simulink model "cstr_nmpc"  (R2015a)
settings: Solver=ode15s  StartTime=0.0  StopTime=5  RelTol=1e-5
StopFcn:
  | plot_reactor
undefined symbols (not defined in the file or in its folder): nmpc
libraries: simulink x4

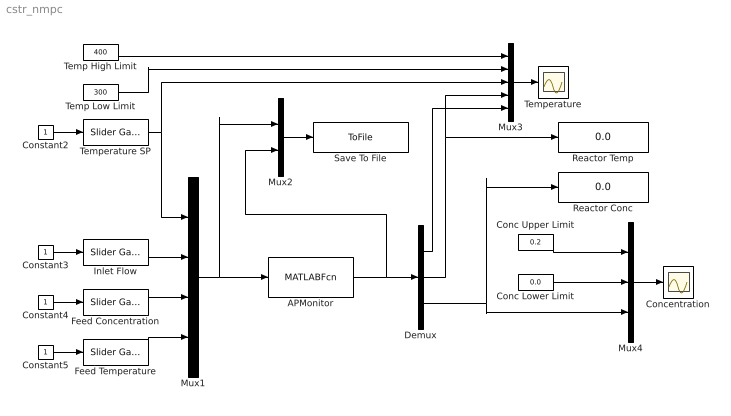
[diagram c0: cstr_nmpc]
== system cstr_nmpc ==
  APMonitor : MATLABFcn  MATLABFcn=nmpc(u)  OutputDimensions=3  SampleTime=0.05
  Conc Lower Limit : Constant  Value=0.0
  Conc Upper Limit : Constant  Value=0.2
  Concentration : Scope
  Constant{2..5} (4 alike) : Constant
  Demux : Demux  Outputs=3
  Feed Concentration : simulink/Math Operations/Slider Gain  low=0  gain=1  high=1
  Feed Temperature : simulink/Math Operations/Slider Gain  low=300  gain=350  high=400
  Inlet Flow : simulink/Math Operations/Slider Gain  low=0  gain=100  high=200
  Mux1 : Mux
  Mux2 : Mux  Inputs=2
  Mux3 : Mux  Inputs=5
  Mux4 : Mux  Inputs=3
  Reactor Conc : Display
  Reactor Temp : Display
  Save To File : ToFile  Filename=data.mat  MatrixName=cstr  SampleTime=0.05
  Temp High Limit : Constant  Value=400
  Temp Low Limit : Constant  Value=300
  Temperature : Scope
  Temperature SP : simulink/Math Operations/Slider Gain  low=300  gain=370  high=400
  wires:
  APMonitor/1 -> Mux2/2, Demux/1
  Constant3/1 -> Inlet Flow/1
  Mux2/1 -> Save To File/1
  Mux1/1 -> Mux2/1, APMonitor/1
  Inlet Flow/1 -> Mux1/2
  Constant2/1 -> Temperature SP/1
  Temperature SP/1 -> Mux1/1, Mux3/3
  Demux/3 -> Reactor Conc/1, Mux4/3
  Constant4/1 -> Feed Concentration/1
  Constant5/1 -> Feed Temperature/1
  Feed Temperature/1 -> Mux1/4
  Temp High Limit/1 -> Mux3/1
  Temp Low Limit/1 -> Mux3/2
  Mux3/1 -> Temperature/1
  Conc Upper Limit/1 -> Mux4/1
  Conc Lower Limit/1 -> Mux4/2
  Mux4/1 -> Concentration/1
  Demux/2 -> Reactor Temp/1, Mux3/4
  Feed Concentration/1 -> Mux1/3
  Demux/1 -> Mux3/5
